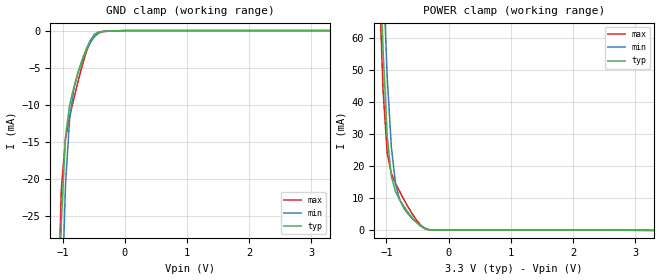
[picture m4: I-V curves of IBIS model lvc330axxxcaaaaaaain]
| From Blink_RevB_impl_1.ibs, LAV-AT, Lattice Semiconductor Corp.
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[Model] lvc330axxxcaaaaaaain
Model_type Input
Polarity   Non-Inverting
Enable   Active-High
Vinl =  0.800V
Vinh =  2.000V
C_comp   5.000pF   4.000pF   5.500pF
[Temperature Range]   25.000   0.125k   -40.000
[Voltage Range]   3.300V   3.140V   3.470V
[C Comp Corner]
C_comp   5.000pF   4.000pF   5.500pF
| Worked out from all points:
|   GND clamp passes 1 mA (typ) near -0.53 V on its own axis
|   POWER clamp passes 1 mA (typ) near -0.42 V on its own axis
[GND_clamp]
|Voltage   I(typ)   I(min)   I(max)
-3.3V     -1.861A    -1.855A    -1.868A
-1.089V   -50.83mA   -68.22mA   -41.82mA
-1.022V   -25.77mA   -39.1mA    -21.38mA
-955mV    -14.31mA   -20.76mA   -14.62mA
-888mV    -10.03mA   -11.87mA   -11.63mA
-821mV    -7.659mA   -7.898mA   -9.194mA
-754mV    -5.715mA   -5.669mA   -6.896mA
-620mV    -2.446mA   -2.675mA   -2.887mA
-486mV    -500.9uA   -793.4uA   -505.6uA
-419mV    -184.7uA   -329.7uA   -182uA
-17mV     -4.77uA    -4.566uA   -5.557uA
3.3V      0A         0A         0A
[POWER_clamp]
|Voltage   I(typ)   I(min)   I(max)
-3.266V   2.002A     2.005A     2.003A
-1.122V   95.84mA    122.3mA    80.76mA
-1.055V   56.43mA    81.12mA    43.86mA
-988mV    29.47mA    48.05mA    24.18mA
-921mV    16.85mA    25.99mA    17.74mA
-854mV    12.14mA    14.61mA    14.7mA
-787mV    9.602mA    9.545mA    12.14mA
-720mV    7.548mA    6.946mA    9.7mA
-519mV    2.524mA    2.531mA    3.31mA
-385mV    541.5uA    789.8uA    641.6uA
-184mV    92.6uA     101.5uA    92.6uA
3.3V      0A         0A         50.77uA
